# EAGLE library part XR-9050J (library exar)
Data SYNCHRONIZER/RLL ENDEC
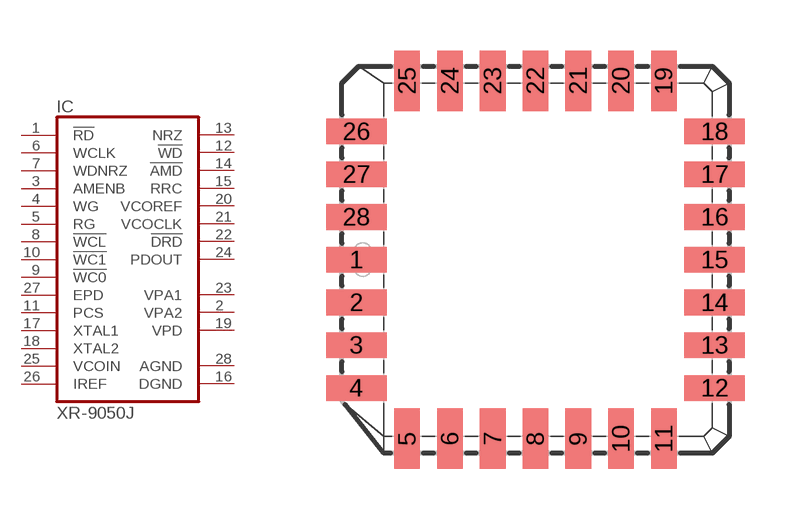
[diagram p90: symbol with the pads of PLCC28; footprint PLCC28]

Designator prefix IC

## XR-9050J (OC_FARNELL: unknown; OC_NEWARK: unknown)  [PLCC28]
1  !RD  in
2  VPA2  pwr
3  AMENB  in
4  WG  in
5  RG  in
6  WCLK  in
7  WDNRZ  in
8  !WCL  in
9  !WC0  in
10  !WC1  in
11  PCS  in
12  !WD  out
13  NRZ
14  !AMD  out
15  RRC  out
16  DGND  pwr
17  XTAL1  in
18  XTAL2  in
19  VPD  pwr
20  VCOREF  out
21  VCOCLK  out
22  !DRD  out
23  VPA1  pwr
24  PDOUT  out
25  VCOIN  in
26  IREF  in
27  EPD  in
28  AGND  pwr

## Footprint PLCC28 (pad centres in mm)
Plastic Leaded Chip Carrier
smd 1.8 x 0.76: 1 -5.32,0; 2 -5.32,-1.27; 3 -5.32,-2.54; 4 -5.32,-3.81; 12 5.32,-3.81; 13 5.32,-2.54; 14 5.32,-1.27; 15 5.32,0; 16 5.32,1.27; 17 5.32,2.54; 18 5.32,3.81; 26 -5.32,3.81; 27 -5.32,2.54; 28 -5.32,1.27
smd 0.76 x 1.8: 5 -3.81,-5.32; 6 -2.54,-5.32; 7 -1.27,-5.32; 8 0,-5.32; 9 1.27,-5.32; 10 2.54,-5.32; 11 3.81,-5.32; 19 3.81,5.32; 20 2.54,5.32; 21 1.27,5.32; 22 0,5.32; 23 -1.27,5.32; 24 -2.54,5.32; 25 -3.81,5.32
